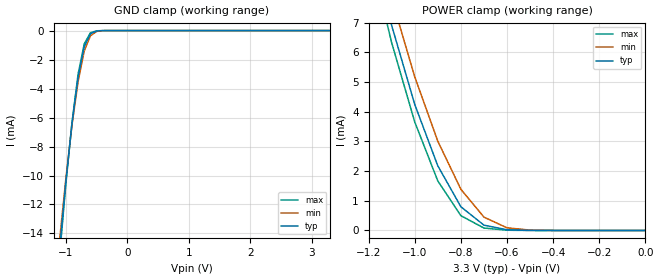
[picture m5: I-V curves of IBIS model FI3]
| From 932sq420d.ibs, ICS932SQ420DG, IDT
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|   Model FI3
[Model]   FI3
Model_type   Input
Polarity   Non-Inverting
Vinl =   0.80V
Vinh =   2.00V
C_comp   3.40pF   2.85pF   3.95pF
[Temperature Range]   27.00   70.00   0.000
[Voltage Range]   3.30V   3.00V   3.70V
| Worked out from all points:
|   GND clamp passes 1 mA (typ) near -0.69 V on its own axis
|   POWER clamp passes 1 mA (typ) near -0.81 V on its own axis
[GND_clamp]
| voltage   I(typ)   I(min)   I(max)
-3.3V     -140mA     -130mA     -150mA
-1.1V     -15.03mA   -14.4mA    -15.5mA
-1V       -10.44mA   -10.23mA   -10.61mA
-900mV    -6.42mA    -6.53mA    -6.34mA
-800mV    -3.2mA     -3.51mA    -2.98mA
-700mV    -1.11mA    -1.4mA     -910uA
-600mV    -220uA     -360uA     -150uA
-500mV    -27.68uA   -59.14uA   -15.29uA
-400mV    -2.43uA    -7.33uA    -1.01uA
3.3V      150pA      140nA      93.85pA
[POWER_clamp]
| voltage   I(typ)   I(min)   I(max)
-3.3V     150mA      140mA      150mA
-1.2V     10.05mA    10.86mA    9.56mA
-1.1V     6.91mA     7.82mA     6.33mA
-1V       4.25mA     5.18mA     3.66mA
-900mV    2.18mA     3.01mA     1.67mA
-800mV    800uA      1.39mA     500uA
-700mV    180uA      450uA      82.19uA
-600mV    23.89uA    89.39uA    8.44uA
-500mV    2.38uA     12.85uA    610nA
0V        150pA      1.12nA     140pA
